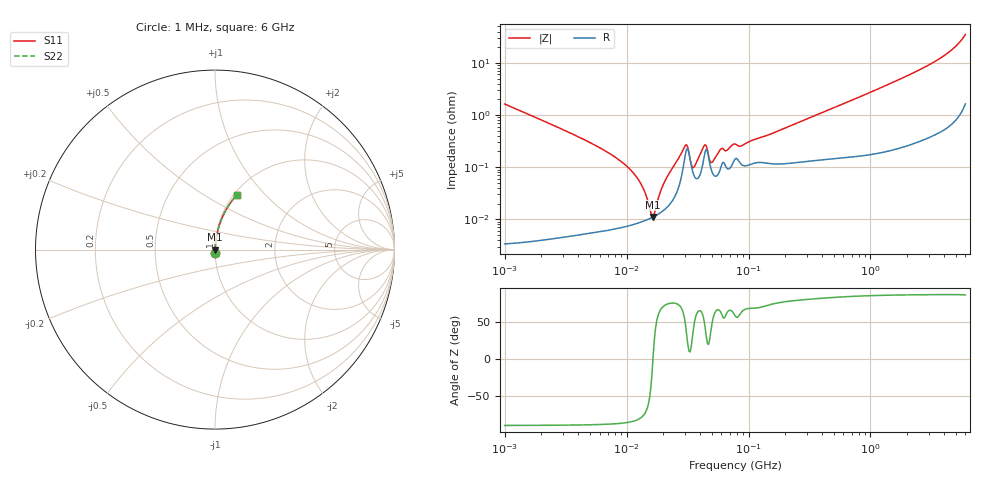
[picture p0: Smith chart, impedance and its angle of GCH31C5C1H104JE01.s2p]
!Murata Part Number: GCH31C5C1H104JE01
!These Parameters are Measured in Series Mode Connection
!Data Generated on Mar 13, 2026
!  o--ll--o
!Port1  Port2
!  o------o
!Operation Temp=25[degC], DC Bias Voltage=0[V]
!Freq. Start=1000[kHz] Stop=6[GHz] 401[Steps]
# Hz S RI R 50
!Freq.(Hz) S11(Real) S11(Imag) S21(Real) S21(Imag) S12(Real) S12(Imag) S22(Real) S22(Imag)
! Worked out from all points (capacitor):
!   401 points, 1 MHz to 6 GHz, reference 50 ohm
!   read as one part in series: C = 97.5 nF near 1.044 MHz
!   lowest |Z| = 11.1 mohm at 16.54 MHz (marker M1)
!   series resonance near 16.45 MHz, so ESL is about 960 pH
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1000000  0.000298 -0.0163  0.9997 0.0163  0.9997 0.0163  0.000298 -0.0163
4293785  6.35e-05 -0.00355  0.9999 0.00355  0.9999 0.00355  6.35e-05 -0.00355
7558231  6.61e-05 -0.00172  0.9999 0.00172  0.9999 0.00172  6.61e-05 -0.00172
1.093935e7  7.79e-05 -0.000852  0.9999 0.000852  0.9999 0.000852  7.79e-05 -0.000852
1.330454e7  8.94e-05 -0.000442  0.9999 0.000442  0.9999 0.000442  8.94e-05 -0.000442
1.583299e7  0.000105 -8.13e-05  0.9999 8.13e-05  0.9999 8.13e-05  0.000105 -8.13e-05
1.653689e7  0.000111 1.08e-05  0.9999 -1.08e-05  0.9999 -1.08e-05  0.000111 1.08e-05
1.843659e7  0.000128 0.000249  0.9999 -0.000249  0.9999 -0.000249  0.000128 0.000249
2.146833e7  0.00017 0.000624  0.9998 -0.000624  0.9998 -0.000624  0.00017 0.000624
3.040356e7  0.00179 0.00193  0.9982 -0.00193  0.9982 -0.00193  0.00179 0.00193
3.175522e7  0.00225 0.000835  0.9977 -0.000835  0.9977 -0.000835  0.00225 0.000835
3.540316e7  0.000728 0.000657  0.9993 -0.000657  0.9993 -0.000657  0.000728 0.000657
4.305766e7  0.00149 0.00204  0.9985 -0.00204  0.9985 -0.00204  0.00149 0.00204
4.497189e7  0.0022 0.00135  0.9978 -0.00135  0.9978 -0.00135  0.0022 0.00135
5.013812e7  0.000819 0.000919  0.9992 -0.000919  0.9992 -0.000919  0.000819 0.000919
5.966657e7  0.00104 0.00201  0.999 -0.00201  0.999 -0.00201  0.00104 0.00201
7.745967e7  0.00143 0.00239  0.9986 -0.00239  0.9986 -0.00239  0.00143 0.00239
8.825674e7  0.00111 0.00233  0.9989 -0.00233  0.9989 -0.00233  0.00111 0.00233
3.325952e8  0.0014 0.00914  0.9986 -0.00914  0.9986 -0.00914  0.0014 0.00914
1.428092e9  0.00359 0.0392  0.9964 -0.0392  0.9964 -0.0392  0.00359 0.0392
3.638376e9  0.0181 0.1157  0.9819 -0.1157  0.9819 -0.1157  0.0181 0.1157
6e9  0.1207 0.3033  0.8793 -0.3033  0.8793 -0.3033  0.1207 0.3033
